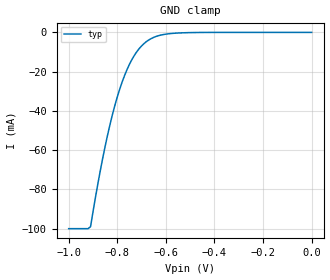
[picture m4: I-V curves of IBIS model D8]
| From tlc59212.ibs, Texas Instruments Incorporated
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|   Model D8
[Model]   D8
Model_type   Input
Vinl = .8
Vinh = 2
|   typ   min   max
C_comp   5.5p   NA   NA
[Voltage Range]   5   NA   NA
[Temperature Range]   27   NA   NA
[Power Clamp Reference]   5   NA   NA
[GND Clamp Reference]   -0   NA   NA
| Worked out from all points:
|   GND clamp passes 1 mA (typ) near -0.61 V on its own axis
[GND Clamp]
|   Voltage   I(typ)   I(min)   I(max)
-1V       -100mA     NA         NA
-910mV    -99.01mA   NA         NA
-880mV    -77.26mA   NA         NA
-850mV    -58.12mA   NA         NA
-820mV    -41.96mA   NA         NA
-800mV    -32.94mA   NA         NA
-770mV    -21.99mA   NA         NA
-740mV    -13.9mA    NA         NA
-680mV    -4.693mA   NA         NA
-630mV    -1.662mA   NA         NA
-550mV    -321.1uA   NA         NA
0V        0A         NA         NA
